(* Logix 5000 AddOnInstructionDefinition export AMCI_NXFE2_Home_CCW; software revision 20.03 *)

ADD_ON_INSTRUCTION AMCI_NXFE2_Home_CCW   (* revision 1.0, vendor AMCI, ExecuteEnableInFalse *)
VAR_INPUT
   Axis_Status_Bits : INT; {required}
   Programmed_Speed : DINT; {required}
   Acceleration : INT; {required}
   Deceleration : INT; {required}
END_VAR
VAR_IN_OUT
   NXFE2_output_data : _000A:NXFE2_0986AEB4:O:0; {required}
END_VAR
VAR_OUTPUT
   EN : BOOL; {access Read Only, visible}
   ER : BOOL; {access Read Only, visible}
END_VAR
VAR
   Upper_Result_X_1000 : DINT;
   command_data_block : INT[10];
        [0]   // Command Bits MSW
        [1]   // Command Bits LSW
        [2]   // Upper Target Position
        [3]   // Lower Target Position
        [4]   // Upper Programmed Speed
        [5]   // Lower Programmed Speed
   index : INT;
END_VAR

ROUTINE EnableInFalse   (* ladder *)
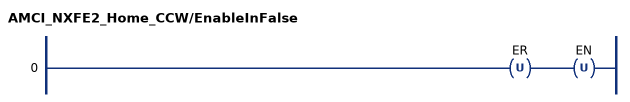
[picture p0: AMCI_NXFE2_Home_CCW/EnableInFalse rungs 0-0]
   0: OTU(ER)OTU(EN);
END_ROUTINE

ROUTINE Logic   (* ladder *)
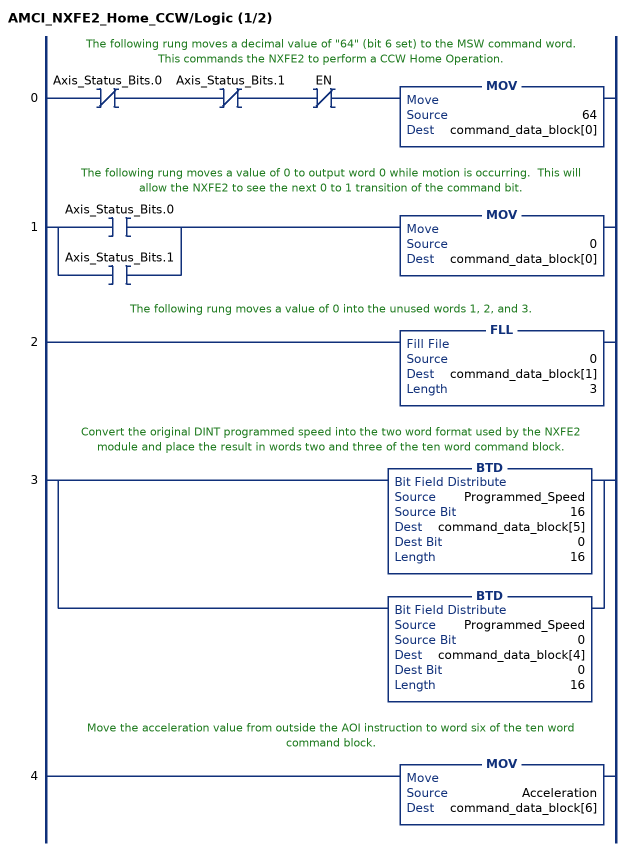
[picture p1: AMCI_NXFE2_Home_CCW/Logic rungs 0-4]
   // The following rung moves a decimal value of "64" (bit 6 set) to the MSW command word.  This commands the NXFE2 to perform a CCW Home Operation.
   0: XIO(Axis_Status_Bits.0)XIO(Axis_Status_Bits.1)XIO(EN)MOV(64,command_data_block[0]);
   // The following rung moves a value of 0 to output word 0 while motion is occurring.  This will allow the NXFE2 to see the next 0 to 1 transition of the command bit.
   1: [XIC(Axis_Status_Bits.0) ,XIC(Axis_Status_Bits.1) ]MOV(0,command_data_block[0]);
   // The following rung moves a value of 0 into the unused words 1, 2, and 3.
   2: FLL(0,command_data_block[1],3);
   // Convert the original DINT programmed speed into the two word format used by the NXFE2 module and place the result in words two and three of the ten word command block.
   3: [BTD(Programmed_Speed,16,command_data_block[5],0,16) ,BTD(Programmed_Speed,0,command_data_block[4],0,16) ];
   // Move the acceleration value from outside the AOI instruction to word six of the ten word command block.
   4: MOV(Acceleration,command_data_block[6]);
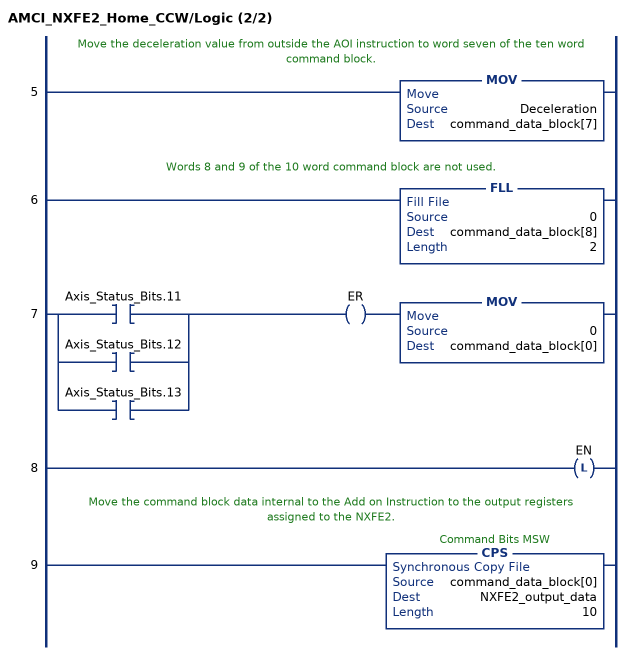
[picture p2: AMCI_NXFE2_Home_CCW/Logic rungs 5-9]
   // Move the deceleration value from outside the AOI instruction to word seven of the ten word command block.
   5: MOV(Deceleration,command_data_block[7]);
   // Words 8 and 9 of the 10 word command block are not used.
   6: FLL(0,command_data_block[8],2);
   7: [XIC(Axis_Status_Bits.11) ,XIC(Axis_Status_Bits.12) ,XIC(Axis_Status_Bits.13) ]OTE(ER)MOV(0,command_data_block[0]);
   8: OTL(EN);
   // Move the command block data internal to the Add on Instruction to the output registers assigned to the NXFE2.
   9: CPS(command_data_block[0],NXFE2_output_data,10);
END_ROUTINE
END_ADD_ON_INSTRUCTION
